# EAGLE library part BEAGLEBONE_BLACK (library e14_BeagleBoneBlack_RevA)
BeagleBone Black Rev. C device with associated package to help create a cape. NOTE: Other considerations when making a Cape (mechanical allowances for tall BBB components, EEPROM requirements, and power ratings) can be found in the BBB System Reference Manual More information available at http://www.element14.com/community/community/designcenter/single-board-computers/next-gen_beaglebone
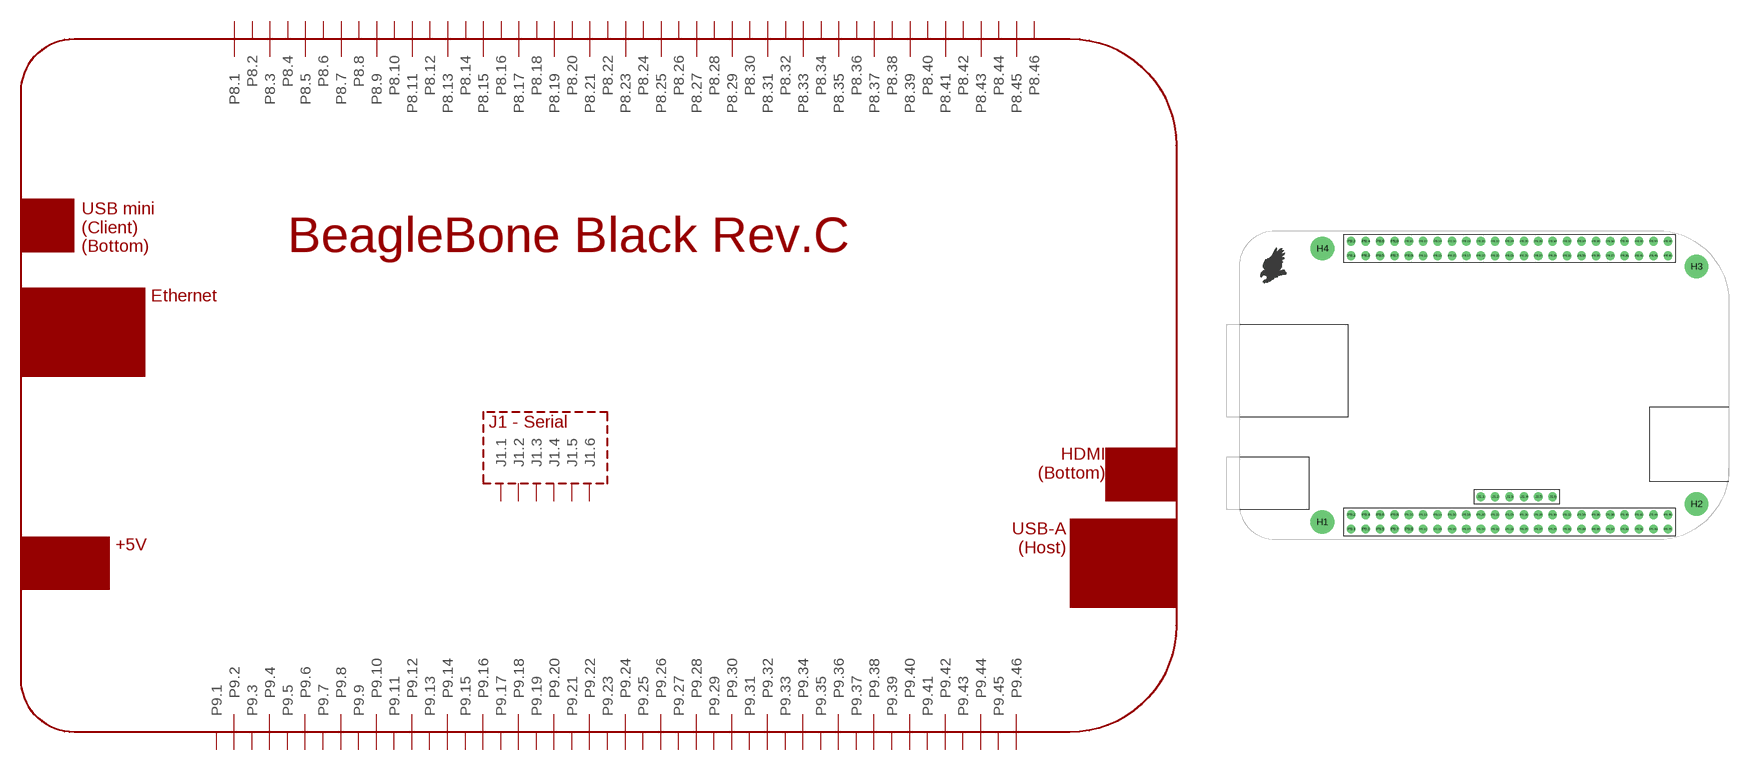
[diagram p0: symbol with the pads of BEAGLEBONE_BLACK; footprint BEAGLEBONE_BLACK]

Designator prefix PCB

## BEAGLEBONE_BLACK  [BEAGLEBONE_BLACK]
J1.1  J1.1
J1.2  J1.2
J1.3  J1.3
J1.4  J1.4
J1.5  J1.5
J1.6  J1.6
P8.1  P8.1
P8.2  P8.2
P8.3  P8.3
P8.4  P8.4
P8.5  P8.5
P8.6  P8.6
P8.7  P8.7
P8.8  P8.8
P8.9  P8.9
P8.10  P8.10
P8.11  P8.11
P8.12  P8.12
P8.13  P8.13
P8.14  P8.14
P8.15  P8.15
P8.16  P8.16
P8.17  P8.17
P8.18  P8.18
P8.19  P8.19
P8.20  P8.20
P8.21  P8.21
P8.22  P8.22
P8.23  P8.23
P8.24  P8.24
P8.25  P8.25
P8.26  P8.26
P8.27  P8.27
P8.28  P8.28
P8.29  P8.29
P8.30  P8.30
P8.31  P8.31
P8.32  P8.32
P8.33  P8.33
P8.34  P8.34
P8.35  P8.35
P8.36  P8.36
P8.37  P8.37
P8.38  P8.38
P8.39  P8.39
P8.40  P8.40
P8.41  P8.41
P8.42  P8.42
P8.43  P8.43
P8.44  P8.44
P8.45  P8.45
P8.46  P8.46
P9.1  P9.1
P9.2  P9.2
P9.3  P9.3
P9.4  P9.4
P9.5  P9.5
P9.6  P9.6
P9.7  P9.7
P9.8  P9.8
P9.9  P9.9
P9.10  P9.10
P9.11  P9.11
P9.12  P9.12
P9.13  P9.13
P9.14  P9.14
P9.15  P9.15
P9.16  P9.16
P9.17  P9.17
P9.18  P9.18
P9.19  P9.19
P9.20  P9.20
P9.21  P9.21
P9.22  P9.22
P9.23  P9.23
P9.24  P9.24
P9.25  P9.25
P9.26  P9.26
P9.27  P9.27
P9.28  P9.28
P9.29  P9.29
P9.30  P9.30
P9.31  P9.31
P9.32  P9.32
P9.33  P9.33
P9.34  P9.34
P9.35  P9.35
P9.36  P9.36
P9.37  P9.37
P9.38  P9.38
P9.39  P9.39
P9.40  P9.40
P9.41  P9.41
P9.42  P9.42
P9.43  P9.43
P9.44  P9.44
P9.45  P9.45
P9.46  P9.46

## Footprint BEAGLEBONE_BLACK (pad centres in mm)
Package for BeagleBone Black Rev. C board.
drill 3.175: H1 14.605,3.175; H2 80.645,6.35; H3 80.645,48.26; H4 14.605,51.435
drill 1.016: J1.1 42.545,7.62; J1.2 45.085,7.62; J1.3 47.625,7.62; J1.4 50.165,7.62; J1.5 52.705,7.62; J1.6 55.245,7.62; P8.1 19.685,50.165; P8.2 19.685,52.705; P8.3 22.225,50.165; P8.4 22.225,52.705; P8.5 24.765,50.165; P8.6 24.765,52.705; P8.7 27.305,50.165; P8.8 27.305,52.705; P8.9 29.845,50.165; P8.10 29.845,52.705; P8.11 32.385,50.165; P8.12 32.385,52.705; P8.13 34.925,50.165; P8.14 34.925,52.705; P8.15 37.465,50.165; P8.16 37.465,52.705; P8.17 40.005,50.165; P8.18 40.005,52.705; P8.19 42.545,50.165; P8.20 42.545,52.705; P8.21 45.085,50.165; P8.22 45.085,52.705; P8.23 47.625,50.165; P8.24 47.625,52.705; P8.25 50.165,50.165; P8.26 50.165,52.705; P8.27 52.705,50.165; P8.28 52.705,52.705; P8.29 55.245,50.165; P8.30 55.245,52.705; P8.31 57.785,50.165; P8.32 57.785,52.705; P8.33 60.325,50.165; P8.34 60.325,52.705; P8.35 62.865,50.165; P8.36 62.865,52.705; P8.37 65.405,50.165; P8.38 65.405,52.705; P8.39 67.945,50.165; P8.40 67.945,52.705; P8.41 70.485,50.165; P8.42 70.485,52.705; P8.43 73.025,50.165; P8.44 73.025,52.705; P8.45 75.565,50.165; P8.46 75.565,52.705; P9.1 19.685,1.905; P9.2 19.685,4.445; P9.3 22.225,1.905; P9.4 22.225,4.445; P9.5 24.765,1.905; P9.6 24.765,4.445; P9.7 27.305,1.905; P9.8 27.305,4.445; P9.9 29.845,1.905; P9.10 29.845,4.445; P9.11 32.385,1.905; P9.12 32.385,4.445; P9.13 34.925,1.905; P9.14 34.925,4.445; P9.15 37.465,1.905; P9.16 37.465,4.445; P9.17 40.005,1.905; P9.18 40.005,4.445; P9.19 42.545,1.905; P9.20 42.545,4.445; P9.21 45.085,1.905; P9.22 45.085,4.445; P9.23 47.625,1.905; P9.24 47.625,4.445; P9.25 50.165,1.905; P9.26 50.165,4.445; P9.27 52.705,1.905; P9.28 52.705,4.445; P9.29 55.245,1.905; P9.30 55.245,4.445; P9.31 57.785,1.905; P9.32 57.785,4.445; P9.33 60.325,1.905; P9.34 60.325,4.445; P9.35 62.865,1.905; P9.36 62.865,4.445; P9.37 65.405,1.905; P9.38 65.405,4.445; P9.39 67.945,1.905; P9.40 67.945,4.445; P9.41 70.485,1.905; P9.42 70.485,4.445; P9.43 73.025,1.905; P9.44 73.025,4.445; P9.45 75.565,1.905; P9.46 75.565,4.445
